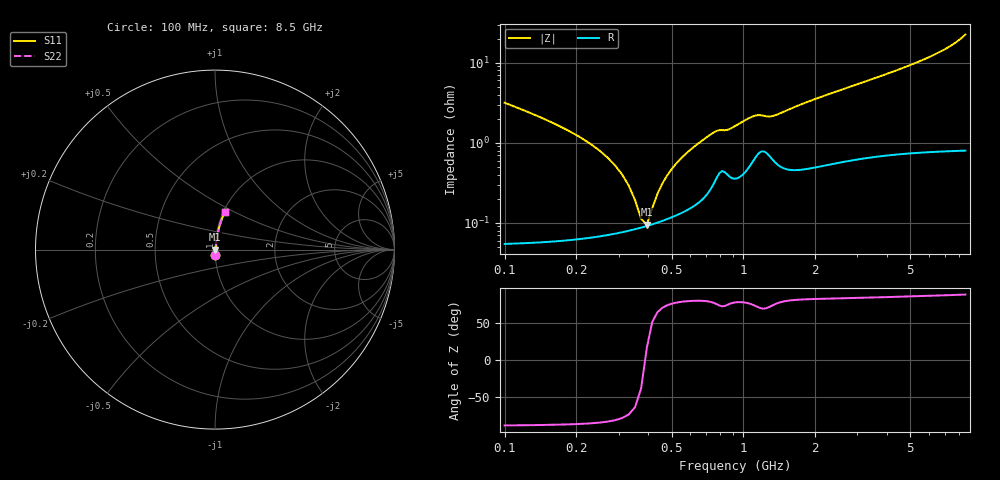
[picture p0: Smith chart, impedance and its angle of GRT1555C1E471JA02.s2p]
!Murata Part Number: GRT1555C1E471JA02
!These Parameters are Measured in Series Mode Connection
!Data Generated on Jun 19, 2026
!  o--ll--o
!Port1  Port2
!  o------o
!Operation Temp=25[degC], DC Bias Voltage=0[V]
!Freq. Start=100[MHz] Stop=9[GHz] 401[Steps]
# Hz S RI R 50
!Freq.(Hz) S11(Real) S11(Imag) S21(Real) S21(Imag) S12(Real) S12(Imag) S22(Real) S22(Imag)
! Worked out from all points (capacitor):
!   401 points, 100 MHz to 8.5 GHz, reference 50 ohm
!   read as one part in series: C = 470 pF near 142 MHz
!   lowest |Z| = 95 mohm at 394 MHz (marker M1)
!   series resonance near 388.3 MHz, so ESL is about 360 pH
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1e8  0.00154 -0.0316  0.9985 0.0316  0.9985 0.0316  0.00154 -0.0316
1.42e8  0.000996 -0.0206  0.999 0.0206  0.999 0.0206  0.000996 -0.0206
2.47e8  0.000739 -0.00816  0.9993 0.00816  0.9993 0.00816  0.000739 -0.00816
2.89e8  0.000757 -0.00523  0.9992 0.00523  0.9992 0.00523  0.000757 -0.00523
3.1e8  0.000777 -0.00396  0.9992 0.00396  0.9992 0.00396  0.000777 -0.00396
3.52e8  0.000834 -0.00171  0.9992 0.00171  0.9992 0.00171  0.000834 -0.00171
3.73e8  0.000871 -0.000698  0.9991 0.000698  0.9991 0.000698  0.000871 -0.000698
3.94e8  0.000912 0.000261  0.9991 -0.000261  0.9991 -0.000261  0.000912 0.000261
4.15e8  0.000958 0.00117  0.999 -0.00117  0.999 -0.00117  0.000958 0.00117
4.78e8  0.00112 0.00369  0.9989 -0.00369  0.9989 -0.00369  0.00112 0.00369
5.41e8  0.00133 0.00598  0.9987 -0.00598  0.9987 -0.00598  0.00133 0.00598
6.25e8  0.00172 0.00887  0.9983 -0.00887  0.9983 -0.00887  0.00172 0.00887
7.3e8  0.0028 0.0124  0.9972 -0.0124  0.9972 -0.0124  0.0028 0.0124
1.108e9  0.00655 0.0205  0.9934 -0.0205  0.9934 -0.0205  0.00655 0.0205
1.318e9  0.00663 0.0203  0.9934 -0.0203  0.9934 -0.0203  0.00663 0.0203
1.507e9  0.00527 0.0244  0.9947 -0.0244  0.9947 -0.0244  0.00527 0.0244
2.074e9  0.00629 0.0359  0.9937 -0.0359  0.9937 -0.0359  0.00629 0.0359
2.914e9  0.0087 0.0511  0.9913 -0.0511  0.9913 -0.0511  0.0087 0.0511
4.3e9  0.013 0.0769  0.987 -0.0769  0.987 -0.0769  0.013 0.0769
5.707e9  0.0192 0.107  0.9808 -0.107  0.9808 -0.107  0.0192 0.107
7.114e9  0.0299 0.1465  0.9701 -0.1465  0.9701 -0.1465  0.0299 0.1465
8.5e9  0.055 0.211  0.945 -0.211  0.945 -0.211  0.055 0.211
